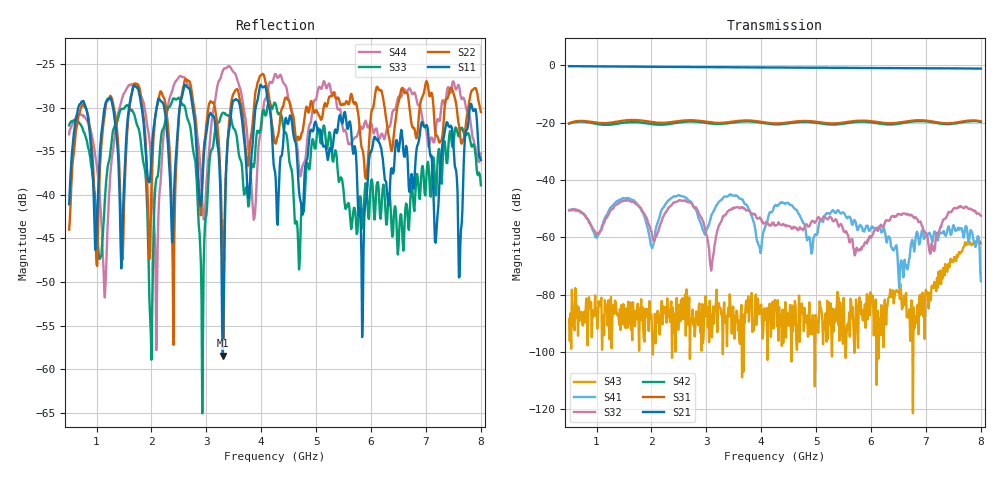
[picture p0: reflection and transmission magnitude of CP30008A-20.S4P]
! Amtery
! Email: info@amtery.com
! Phone: 886-2-2883-7839
! Model Number: CP30008A-20
! 4-port S-parameter measurement data for Dual-Directional Coupler
! Frequency Range: 0.5 GHz to 8 GHz
! Port 1: Input
! Port 2: Output
! Port 3: Coupled Forward
! Port 4: Coupled Reverse
# Hz S dB R 50
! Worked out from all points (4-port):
!   601 points, 500 MHz to 8 GHz, reference 50 ohm
!   strongest paths, dB at 500 MHz, 2.375 GHz, 4.25 GHz, 6.125 GHz, 8 GHz:
!     S21: -0.2, -0.5, -0.7, -0.9, -1.1
!     S31: -20.2, -19.7, -20.2, -19.8, -19.5
!     S42: -20.3, -20.2, -20.6, -20.2, -19.7
!     S32: -50.6, -48.5, -55.9, -57.7, -52.4
!     S41: -50.4, -46.1, -48.8, -56.5, -75.2
!     S43: -88.5, -102.0, -81.8, -85.6, -62.0
!   lowest |S11| = -58.5 dB at 3.3 GHz (marker M1), VSWR 1.00, Z = 49.9 - j0.0653 ohm
!   |S11| at or under -10 dB: start of sweep to end of sweep
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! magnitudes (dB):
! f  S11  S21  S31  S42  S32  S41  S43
! 500 MHz  -41.1  -0.2  -20.2  -20.3  -50.6  -50.4  -88.5
! 1.15 GHz  -30.0  -0.3  -20.1  -20.7  -54.2  -53.3  -81.9
! 1.675 GHz  -27.5  -0.4  -19.0  -19.7  -47.6  -47.0  -86.9
! 1.988 GHz  -37.1  -0.5  -19.7  -20.4  -57.6  -62.5  -87.0
! 3.3 GHz  -58.5  -0.6  -20.0  -20.3  -52.7  -46.3  -100.7
! 4.013 GHz  -27.6  -0.7  -19.7  -20.0  -54.7  -61.1  -89.9
! 8 GHz  -36.0  -1.1  -19.5  -19.7  -52.4  -75.2  -62.0
